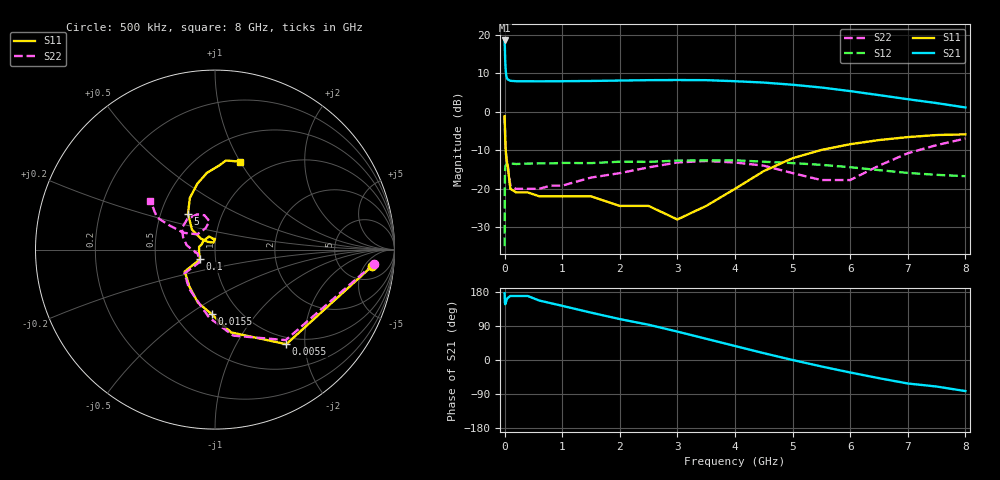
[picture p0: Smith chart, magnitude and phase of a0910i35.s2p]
!  MSA-0910 S AND NOISE PARAMETERS
!  Id=35mA  LAST UPDATED 07-27-92
# ghz s ma r 50
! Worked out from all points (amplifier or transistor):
!   28 points, 500 kHz to 8 GHz, reference 50 ohm
!   highest |S21| = 18.5 dB at 500 kHz (marker M1)
!   |S21| within 3 dB of that: start of sweep to 6.768 MHz
!   unconditionally stable (mu >= 1): 32.14 MHz to end of sweep
!   at 20.5 MHz: K = 0.85, MSG = 12.2 dB, |S12| = -13.9 dB
!   at 1.5 GHz: K = 1.18, MAG = 8.1 dB, |S12| = -13.3 dB
!   at 8 GHz: K = 1.63, MAG = 4.3 dB, |S12| = -16.7 dB
!   lowest NFmin = 6.00 dB at 100 MHz
!   S11 on the Smith chart (normalised r, x): 500 kHz: 9, -8; 5.5 MHz: 0.88, -1.64; 15.5 MHz: 0.75, -0.62; 100 MHz: 0.84, -0.09; 5 GHz: 0.69, +0.29; 8 GHz: 0.76, +1.00
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0.0005  0.88 -6.0  8.46 176.0  0.018 48.0  0.89 -5.0
0.0055  0.66 -53.0  6.48 153.0  0.14 44.0  0.64 -52.0
0.0105  0.47 -79.0  4.75 147.0  0.184 29.0  0.49 -78.0
0.0155  0.36 -93.0  3.86 148.0  0.199 21.0  0.38 -95.0
0.0205  0.31 -108.0  3.38 151.0  0.202 16.0  0.31 -107.0
0.0305  0.25 -125.0  2.94 156.0  0.207 11.0  0.26 -124.0
0.0405  0.22 -136.0  2.74 160.0  0.209 8.0  0.23 -134.0
0.1  0.1 -147.0  2.53 169.0  0.214 2.0  0.11 -141.0
0.4  0.09 170.0  2.5 169.0  0.213 -1.0  0.1 -167.0
0.6  0.08 159.0  2.49 157.0  0.214 -3.0  0.1 -169.0
1.5  0.08 114.0  2.52 125.0  0.216 -10.0  0.14 176.0
2  0.06 99.0  2.55 108.0  0.225 -14.0  0.16 171.0
2.5  0.06 90.0  2.58 93.0  0.224 -17.0  0.19 159.0
3  0.04 102.0  2.59 75.0  0.233 -22.0  0.22 147.0
3.5  0.06 134.0  2.58 56.0  0.234 -27.0  0.23 132.0
4  0.1 142.0  2.5 37.0  0.235 -35.0  0.22 117.0
4.5  0.17 139.0  2.4 18.0  0.225 -42.0  0.2 107.0
5  0.25 127.0  2.25 0.0  0.216 -49.0  0.16 101.0
5.5  0.32 116.0  2.07 -17.0  0.205 -55.0  0.13 114.0
6  0.38 105.0  1.86 -33.0  0.191 -60.0  0.13 139.0
7  0.47 87.0  1.46 -62.0  0.161 -66.0  0.29 152.0
8  0.51 74.0  1.14 -82.0  0.146 -63.0  0.45 143.0
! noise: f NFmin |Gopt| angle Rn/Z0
0.1  6  0.11  25  1.02
0.5  6  0.09  12  1.03
1  6  0.09  15  1.03
2  6.1  0.05  15  1.03
3  6.3  0.03  -14  1.05
4  6.5  0.05  -71  1.12
